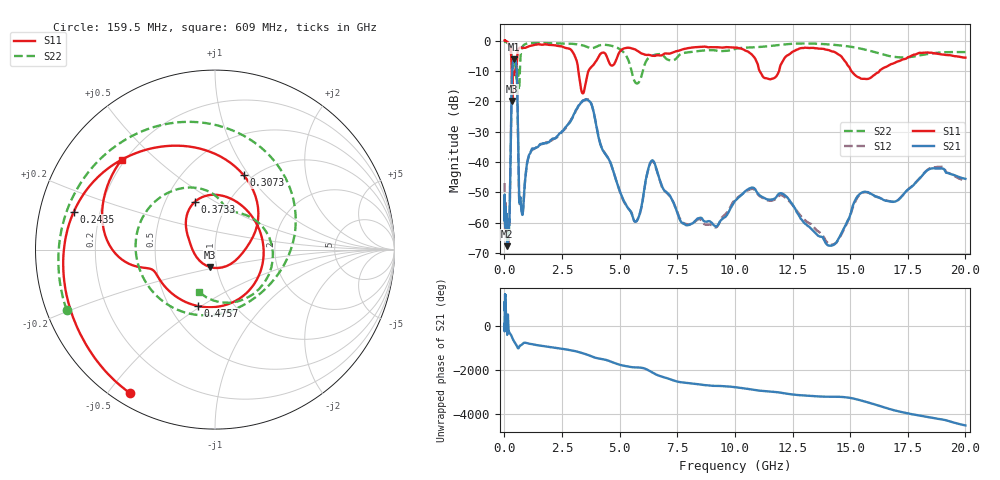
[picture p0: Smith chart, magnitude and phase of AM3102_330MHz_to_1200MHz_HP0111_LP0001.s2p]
! Date/Time: Tue, Sep 11, 2018 5:15 PM
! Network Analyzer: Agilent Technologies E8362B Rev: A.07.50.63
! Sweep from 0.010 to 20.000 GHz, 1601 Points, Sweep Type: LOG
! Power Supply: 4.949 V, 0.001 A
# Hz S DB R 50
!freq MagS11 AngS11 MagS21 AngS21 MagS12 AngS12 MagS22 AngS22
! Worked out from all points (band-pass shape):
!   1601 points, 10 MHz to 20 GHz, reference 50 ohm
!   highest |S21| = -6.17 dB at 426.5 MHz (marker M1); lowest = -67.7 dB at 117.1 MHz (marker M2)
!   |S21| within 3 dB of the highest: 345.3 MHz to 528.3 MHz (183 MHz wide, 41.9 % of centre)
!   lowest |S11| = -19.9 dB at 341.1 MHz (marker M3), VSWR 1.23, Z = 46.3 - j9.05 ohm
!   |S11| at or under -10 dB: 3.208 GHz to 3.65 GHz (441.5 MHz wide, 12.9 % of centre); 11.07 GHz to 11.92 GHz (845.5 MHz wide, 7.36 % of centre); 15.05 GHz to 16.28 GHz (1.231 GHz wide, 7.86 % of centre)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
!   |S22| runs from -16.2 to -0.2 dB; largest |S21 - S12| = 0.0064
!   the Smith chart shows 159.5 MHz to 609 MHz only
!   S11 on the Smith chart (normalised r, x): 159.5 MHz: 0.05, -0.57; 243.5 MHz: 0.10, +0.13; 307.3 MHz: 0.91, +0.94; 373.3 MHz: 0.70, +0.40; 475.7 MHz: 0.69, -0.48; 609 MHz: 0.19, +0.39
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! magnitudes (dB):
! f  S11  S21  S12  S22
! 10 MHz  0.0  -53.1  -46.9  -0.2
! 35.55 MHz  0.0  -60.0  -59.8  -0.4
! 117.1 MHz  -0.4  -67.7  -63.2  -0.7
! 126.4 MHz  -0.4  -64.7  -65.5  -0.8
! 159.5 MHz  -0.6  -64.4  -66.7  -1.0
! 243.5 MHz  -1.8  -51.0  -50.7  -1.9
! 307.3 MHz  -7.0  -19.7  -19.7  -4.9
! 341.1 MHz  -19.9  -9.8  -9.8  -8.7
! 373.3 MHz  -10.8  -7.1  -7.2  -8.6
! 426.5 MHz  -11.3  -6.2  -6.2  -7.1
! 447.2 MHz  -10.6  -6.2  -6.3  -7.1
! 475.7 MHz  -9.7  -6.4  -6.5  -7.9
! 609 MHz  -2.8  -39.6  -39.6  -12.0
! 779.7 MHz  -2.5  -57.4  -57.3  -2.1
! 1.59 GHz  -1.4  -34.0  -34.1  -0.8
! 3.634 GHz  -10.3  -19.6  -19.4  -2.3
! 5.652 GHz  -2.9  -59.6  -59.5  -13.5
! 6.426 GHz  -5.0  -39.4  -39.7  -5.0
! 7.845 GHz  -2.7  -60.6  -60.3  -4.0
! 10.73 GHz  -4.6  -48.4  -48.8  -2.3
! 14.07 GHz  -3.2  -67.5  -66.9  -1.3
! 20 GHz  -5.6  -45.5  -46.4  -3.8
